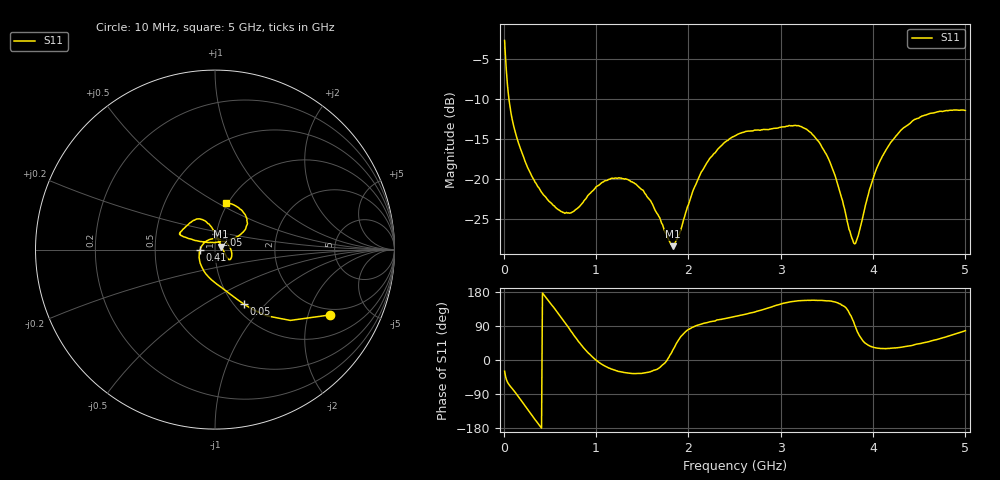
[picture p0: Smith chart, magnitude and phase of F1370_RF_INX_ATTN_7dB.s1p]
! S-parameters for RF_INX input IDT F1370 DPD Demodulator
! Date Measured:  2015-11-25  RGG
!  Port 1 = Pin 35 = RF_INX
! STATE: RF_INX selected, 7 dB attenuation (Gain = Gmax - 7 dB)
! RF Frequency:  10 MHz to 5000 MHz
! RF_INY, IF_I+, IF_I-, IF_Q+, and IF_Q- terminated
! 2300 MHz, 0 dBm signal applied to LO_IN
! Vcc = +5.00 Volts  Icc = approx 275 mA.
! NOTES:  The device was measured on a custom printed circuit evaluation board with individual 50 ohm
!  microstrip lines to the RF and LO pins. The 50 ohm microstrip lines were de-embedded using reference
!  plane extensions
! Instrument Manufacturer:  Agilent Technologies
! Instrument Model:  E5071C
! Instrument Serial Number:  MY46419053
! Instrument Firmware Rev:  A.11.31
! Frequency Re{S11} Im{S11}
# HZ  S  RI R 50.00
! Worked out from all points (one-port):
!   500 points, 10 MHz to 5 GHz, reference 50 ohm
!   lowest |S11| = -28.4 dB at 1.83 GHz (marker M1), VSWR 1.08, Z = 53.5 + j1.76 ohm
!   |S11| at or under -10 dB: 57.14 MHz to end of sweep
!   S11 on the Smith chart (normalised r, x): 10 MHz: 1.75, -2.78; 50 MHz: 1.11, -0.76; 410 MHz: 0.85, -0.00; 2.05 GHz: 1.00, +0.17; 5 GHz: 0.97, +0.55
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1e7  0.6399 -0.3642
5e7  0.1598 -0.3031
9e7  0.0632 -0.2313
1.6e8  -0.0208 -0.1672
2.7e8  -0.0798 -0.0826
4.1e8  -0.0827 -0.000138
6.4e8  -0.0178 0.0593
7.5e8  0.0228 0.0584
9.4e8  0.0797 0.0185
1.08e9  0.0932 -0.023
1.26e9  0.0872 -0.0518
1.52e9  0.069 -0.0464
1.83e9  0.0344 0.0164
1.89e9  0.0274 0.035
2.05e9  0.00473 0.0846
2.23e9  -0.0249 0.1322
2.51e9  -0.0796 0.1694
3.13e9  -0.194 0.0928
3.31e9  -0.1829 0.0763
3.5e9  -0.1284 0.0576
3.61e9  -0.0845 0.0457
3.76e9  -0.0203 0.0399
3.82e9  0.00663 0.0407
3.98e9  0.0751 0.054
4.09e9  0.1161 0.0681
4.38e9  0.1749 0.131
4.69e9  0.1546 0.2123
5e9  0.0589 0.2622
